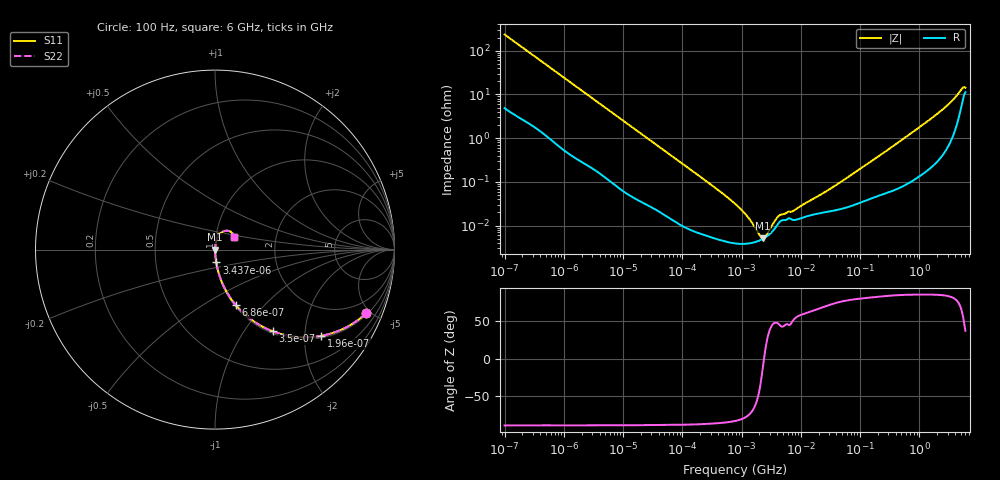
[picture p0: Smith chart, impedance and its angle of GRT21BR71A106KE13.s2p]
!Murata Part Number: GRT21BR71A106KE13
!These Parameters are Measured in Series Mode Connection
!Data Generated on Jun 19, 2026
!  o--ll--o
!Port1  Port2
!  o------o
!Operation Temp=25[degC], DC Bias Voltage=0[V]
!Freq. Start=100[Hz] Stop=6[GHz] 401[Steps]
# Hz S RI R 50
!Freq.(Hz) S11(Real) S11(Imag) S21(Real) S21(Imag) S12(Real) S12(Imag) S22(Real) S22(Imag)
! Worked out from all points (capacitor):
!   401 points, 100 Hz to 6 GHz, reference 50 ohm
!   read as one part in series: C = 6.74 uF near 109 Hz
!   lowest |Z| = 5.06 mohm at 2.269 MHz (marker M1)
!   series resonance near 2.391 MHz, so ESL is about 660 pH
!   S11 on the Smith chart (normalised r, x): 100 Hz: 1.10, -4.71; 196 Hz: 1.05, -2.42; 350 Hz: 1.03, -1.37; 686 Hz: 1.02, -0.71; 3.437 kHz: 1.00, -0.14; 6 GHz: 1.22, +0.17
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100  0.842 -0.3545  0.158 0.3545  0.158 0.3545  0.842 -0.3545
196  0.5929 -0.4803  0.4071 0.4803  0.4071 0.4803  0.5929 -0.4803
350  0.3225 -0.4556  0.6775 0.4556  0.6775 0.4556  0.3225 -0.4556
686  0.1163 -0.3096  0.8837 0.3096  0.8837 0.3096  0.1163 -0.3096
2008  0.0174 -0.1197  0.9826 0.1197  0.9826 0.1197  0.0174 -0.1197
3437  0.00693 -0.0714  0.9931 0.0714  0.9931 0.0714  0.00693 -0.0714
40335  0.000249 -0.00637  0.9998 0.00637  0.9998 0.00637  0.000249 -0.00637
345986  5.16e-05 -0.000756  0.9999 0.000756  0.9999 0.000756  5.16e-05 -0.000756
774597  3.9e-05 -0.000313  1 0.000313  1 0.000313  3.9e-05 -0.000313
1108252  3.81e-05 -0.000192  1 0.000192  1 0.000192  3.81e-05 -0.000192
1585629  4.08e-05 -9.58e-05  1 9.58e-05  1 9.58e-05  4.08e-05 -9.58e-05
2268635  4.92e-05 -1.19e-05  1 1.19e-05  1 1.19e-05  4.92e-05 -1.19e-05
3103719  6.68e-05 5.93e-05  0.9999 -5.93e-05  0.9999 -5.93e-05  6.68e-05 5.93e-05
4440638  0.000123 0.000122  0.9999 -0.000122  0.9999 -0.000122  0.000123 0.000122
7599586  0.000134 0.000173  0.9999 -0.000173  0.9999 -0.000173  0.000134 0.000173
1.555665e7  0.000175 0.000355  0.9998 -0.000355  0.9998 -0.000355  0.000175 0.000355
3.983537e7  0.000226 0.000822  0.9998 -0.000822  0.9998 -0.000822  0.000226 0.000822
3.124326e8  0.000615 0.00567  0.9994 -0.00567  0.9994 -0.00567  0.000615 0.00567
1.565993e9  0.00285 0.0275  0.9971 -0.0275  0.9971 -0.0275  0.00285 0.0275
3.352442e9  0.0122 0.0636  0.9878 -0.0636  0.9878 -0.0636  0.0122 0.0636
5.245841e9  0.0697 0.1054  0.9303 -0.1054  0.9303 -0.1054  0.0697 0.1054
6e9  0.1064 0.0691  0.8936 -0.0691  0.8936 -0.0691  0.1064 0.0691
